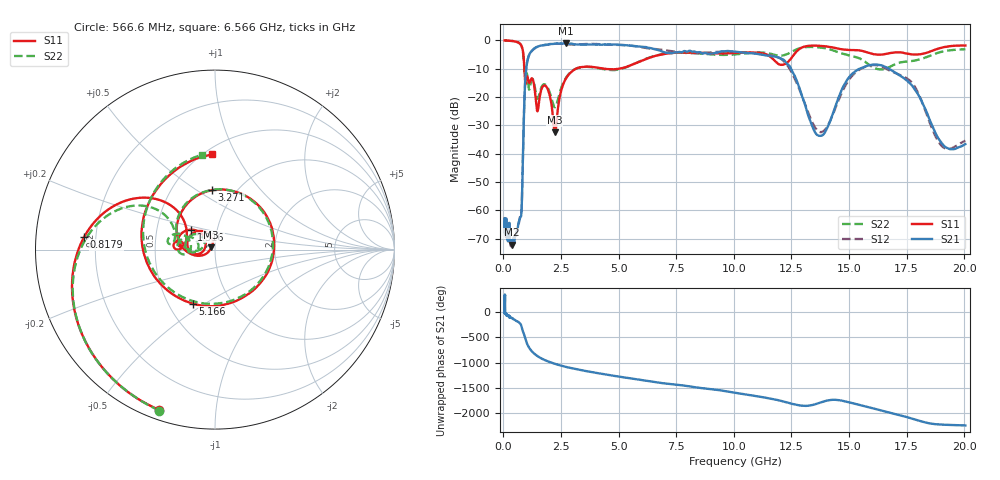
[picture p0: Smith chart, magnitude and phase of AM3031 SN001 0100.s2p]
# Hz S DB R 50
!freq MagS11 AngS11 MagS21 AngS21 MagS12 AngS12 MagS22 AngS22
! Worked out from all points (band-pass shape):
!   1601 points, 50 MHz to 20.05 GHz, reference 50 ohm
!   highest |S21| = -1.05 dB at 2.702 GHz (marker M1); lowest = -72.1 dB at 364.1 MHz (marker M2)
!   |S21| within 3 dB of the highest: 1.192 GHz to 6.93 GHz (5.738 GHz wide, 141 % of centre); 9.397 GHz to 10.16 GHz (758.1 MHz wide, 7.75 % of centre)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
!   lowest |S11| = -32.4 dB at 2.232 GHz (marker M3), VSWR 1.05, Z = 48 + j1.14 ohm
!   |S11| at or under -10 dB: 907.2 MHz to 3.139 GHz (2.232 GHz wide, 110 % of centre); 4.399 GHz to 4.995 GHz (596 MHz wide, 12.7 % of centre)
!   |S22| runs from -23.6 to 0.0 dB; largest |S21 - S12| = 0.067
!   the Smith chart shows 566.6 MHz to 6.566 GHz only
!   S11 on the Smith chart (normalised r, x): 566.6 MHz: 0.04, -0.71; 817.9 MHz: 0.16, +0.05; 1.316 GHz: 0.75, +0.17; 3.271 GHz: 0.78, +0.58; 5.166 GHz: 0.66, -0.45; 6.566 GHz: 0.55, +0.81
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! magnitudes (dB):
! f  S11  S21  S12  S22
! 50 MHz  0.0  -66.0  -62.4  0.0
! 135.9 MHz  0.0  -68.4  -67.7  0.0
! 364.1 MHz  -0.2  -72.1  -71.4  -0.2
! 369.6 MHz  -0.2  -71.5  -71.1  -0.2
! 566.6 MHz  -0.5  -67.9  -67.8  -0.5
! 817.9 MHz  -2.7  -51.1  -50.9  -2.8
! 915.2 MHz  -11.3  -19.6  -19.5  -11.4
! 1.005 GHz  -13.1  -8.9  -8.7  -11.5
! 1.316 GHz  -15.2  -3.0  -3.0  -14.7
! 1.473 GHz  -25.0  -2.2  -2.2  -20.6
! 1.9 GHz  -16.8  -1.5  -1.5  -16.4
! 2.232 GHz  -32.4  -1.1  -1.2  -23.6
! 2.702 GHz  -13.6  -1.1  -1.3  -13.3
! 2.722 GHz  -13.3  -1.1  -1.3  -13.1
! 3.271 GHz  -9.6  -1.4  -1.4  -9.6
! 5.166 GHz  -9.8  -1.6  -1.6  -9.9
! 6.566 GHz  -5.5  -3.1  -3.1  -5.5
! 7.402 GHz  -4.4  -4.3  -3.9  -4.4
! 11.91 GHz  -8.2  -6.0  -6.0  -5.3
! 13.73 GHz  -1.9  -33.7  -32.3  -2.5
! 16.38 GHz  -5.0  -8.8  -9.1  -10.2
! 20.05 GHz  -1.8  -36.6  -35.4  -3.1
